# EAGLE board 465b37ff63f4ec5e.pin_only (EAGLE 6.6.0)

Size 58.42 x 73.66 mm. Coordinates in mm from the lower left corner, seen from the top.
Outline: 0,0 0,12.7 arc-90 2.54,15.24 16.51,15.24 arc90 19.05,17.78 19.05,71.12 arc-90 21.59,73.66 36.83,73.66 arc-90 39.37,71.12 39.37,17.78 arc90 41.91,15.24 55.88,15.24 arc-90 58.42,12.7 58.42,0 0,0
Copper layers (1*16): Top 0.035mm / dielectric 1.5mm / Bottom 0.035mm
Design rules "default": minimum track width 8mil, minimum drill 0.4mm, track to track 8mil, track to pad 8mil, pad to pad 8mil, via to via 8mil, smd to smd 8mil, copper to edge 20mil, drill to drill 8mil, minimum pad ring 8mil, minimum via ring 10mil, stop-mask expansion 3mil, vias tented up to drill 0mil, thermal gap 8mil

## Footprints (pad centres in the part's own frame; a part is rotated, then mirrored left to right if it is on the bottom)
1X20_ROUND = drill 1 pad 1.676 square: 1 -24.13,0 | drill 1 pad 1.676: 2 -21.59,0; 3 -19.05,0; 4 -16.51,0; 5 -13.97,0; 6 -11.43,0; 7 -8.89,0; 8 -6.35,0; 9 -3.81,0; 10 -1.27,0; 11 1.27,0; 12 3.81,0; 13 6.35,0; 14 8.89,0; 15 11.43,0; 16 13.97,0; 17 16.51,0; 18 19.05,0; 19 21.59,0; 20 24.13,0
MOUNTINGHOLE_2.5_PLATED_THICK = drill 2.5 pad 4: P$1 0,0
RASPBERRYPI_B+_IDC = drill 1 pad 1.676 square: 1 -1.27,24.13 | drill 1 pad 1.676: 2 1.27,24.13; 3 -1.27,21.59; 4 1.27,21.59; 5 -1.27,19.05; 6 1.27,19.05; 7 -1.27,16.51; 8 1.27,16.51; 9 -1.27,13.97; 10 1.27,13.97; 11 -1.27,11.43; 12 1.27,11.43; 13 -1.27,8.89; 14 1.27,8.89; 15 -1.27,6.35; 16 1.27,6.35; 17 -1.27,3.81; 18 1.27,3.81; 19 -1.27,1.27; 20 1.27,1.27; 21 -1.27,-1.27; 22 1.27,-1.27; 23 -1.27,-3.81; 24 1.27,-3.81; 25 -1.27,-6.35; 26 1.27,-6.35; 27 -1.27,-8.89; 28 1.27,-8.89; 29 -1.27,-11.43; 30 1.27,-11.43; 31 -1.27,-13.97; 32 1.27,-13.97; 33 -1.27,-16.51; 34 1.27,-16.51; 35 -1.27,-19.05; 36 1.27,-19.05; 37 -1.27,-21.59; 38 1.27,-21.59; 39 -1.27,-24.13; 40 1.27,-24.13

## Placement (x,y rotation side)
JP1  [1X20_ROUND]  36.83,41.91 90 top
JP2  [1X20_ROUND]  21.59,41.91 90 top
U$1  MOUNTINGHOLE2.5_THICK  [MOUNTINGHOLE_2.5_PLATED_THICK]  21.59,71.12 0 top
U$2  MOUNTINGHOLE2.5_THICK  [MOUNTINGHOLE_2.5_PLATED_THICK]  2.54,12.7 0 top
U$3  MOUNTINGHOLE2.5_THICK  [MOUNTINGHOLE_2.5_PLATED_THICK]  36.83,71.12 0 top
U$4  MOUNTINGHOLE2.5_THICK  [MOUNTINGHOLE_2.5_PLATED_THICK]  55.88,12.7 0 top
U$5  [ADAFRUIT_5MM]  27.18,67.06 0 top
X1  [RASPBERRYPI_B+_IDC]  29.21,5.08 90 top

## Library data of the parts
JP1 JP2 U$5 X1 = microbuilder
U$1-U$4 = microbuilder; BOM: EXCLUDE

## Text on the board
tPlace: GPIO21 | GND | GPIO20 | GPIO26 | GPIO16 | GPIO19 | GND | GPIO13 | GPIO12 | GPIO6 | GND | GPIO5 | EECLK | EEDATA | SPICS1 | GND | SPICS0 | SPISCLK | GPIO25 | SPIMISO | GND | SPIMOSI | GPIO24 | 3V3 | GPIO23 | GPIO22 | GND | GPIO27 | GPIO18 | GPIO17 | RXD0 | GND | TXD0 | GPIO4 | GND | SCL1 | 5V0 | SDA1 | 5V0 | 3V3

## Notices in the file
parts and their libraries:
microbuilder: This work is placed in the public domain, and may be freely used for commercial and non-commercial work with the following conditions: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
